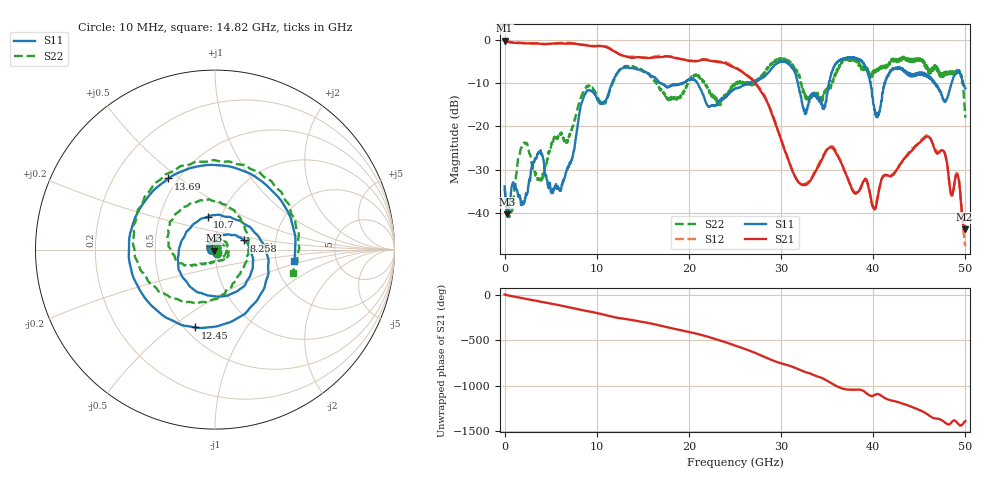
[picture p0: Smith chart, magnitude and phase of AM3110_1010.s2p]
# Hz S DB R 50.0
!freq dBS11 angS11 dBS21 angS21 dBS12 angS12 dBS22 angS22
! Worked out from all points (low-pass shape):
!   1601 points, 10 MHz to 50 GHz, reference 50 ohm
!   highest |S21| = -0.13 dB at 10 MHz (marker M1); lowest = -43.8 dB at 49.91 GHz (marker M2)
!   |S21| within 3 dB of the highest: start of sweep to 12.32 GHz
!   lowest |S11| = -40.4 dB at 291.2 MHz (marker M3), VSWR 1.02, Z = 49.3 - j0.594 ohm
!   |S11| at or under -10 dB: start of sweep to 11.66 GHz; 20.93 GHz to 26.58 GHz (5.651 GHz wide, 23.8 % of centre); 31.84 GHz to 35.19 GHz (3.35 GHz wide, 10 % of centre)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
!   |S22| runs from -41.0 to -3.9 dB; largest |S21 - S12| = 0.029
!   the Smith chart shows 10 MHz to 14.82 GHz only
!   S11 on the Smith chart (normalised r, x): 10 MHz: 1.02, -0.04; 8.258 GHz: 1.38, +0.15; 10.7 GHz: 0.86, +0.33; 12.45 GHz: 0.56, -0.61; 13.69 GHz: 0.45, +0.46; 14.82 GHz: 2.54, -0.39
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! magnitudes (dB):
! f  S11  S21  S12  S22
! 10 MHz  -33.9  -0.1  -0.1  -34.4
! 291.2 MHz  -40.4  -0.4  -0.3  -39.7
! 2.072 GHz  -37.9  -0.7  -0.6  -23.9
! 3.79 GHz  -25.9  -0.8  -0.8  -31.8
! 6.071 GHz  -34.6  -0.8  -0.6  -21.8
! 8.258 GHz  -15.4  -1.1  -1.0  -13.4
! 8.352 GHz  -14.6  -1.1  -1.0  -12.9
! 10.7 GHz  -14.6  -1.4  -1.3  -14.8
! 12.45 GHz  -7.0  -3.3  -3.2  -7.0
! 13.69 GHz  -6.5  -4.1  -3.9  -6.2
! 14.82 GHz  -7.0  -4.0  -4.0  -6.9
! 16.69 GHz  -9.5  -3.9  -3.6  -10.7
! 25 GHz  -11.3  -6.4  -6.3  -10.2
! 33.35 GHz  -12.6  -32.0  -31.8  -13.1
! 35.5 GHz  -7.5  -24.9  -24.5  -10.3
! 38 GHz  -4.0  -35.3  -35.5  -4.4
! 40.47 GHz  -17.9  -36.7  -36.3  -7.0
! 41.69 GHz  -7.8  -31.4  -31.4  -5.9
! 46.03 GHz  -8.6  -22.4  -22.1  -6.5
! 49.19 GHz  -7.3  -31.5  -31.2  -6.9
! 49.91 GHz  -10.9  -43.8  -46.5  -15.0
! 50 GHz  -11.2  -43.2  -47.7  -18.0
